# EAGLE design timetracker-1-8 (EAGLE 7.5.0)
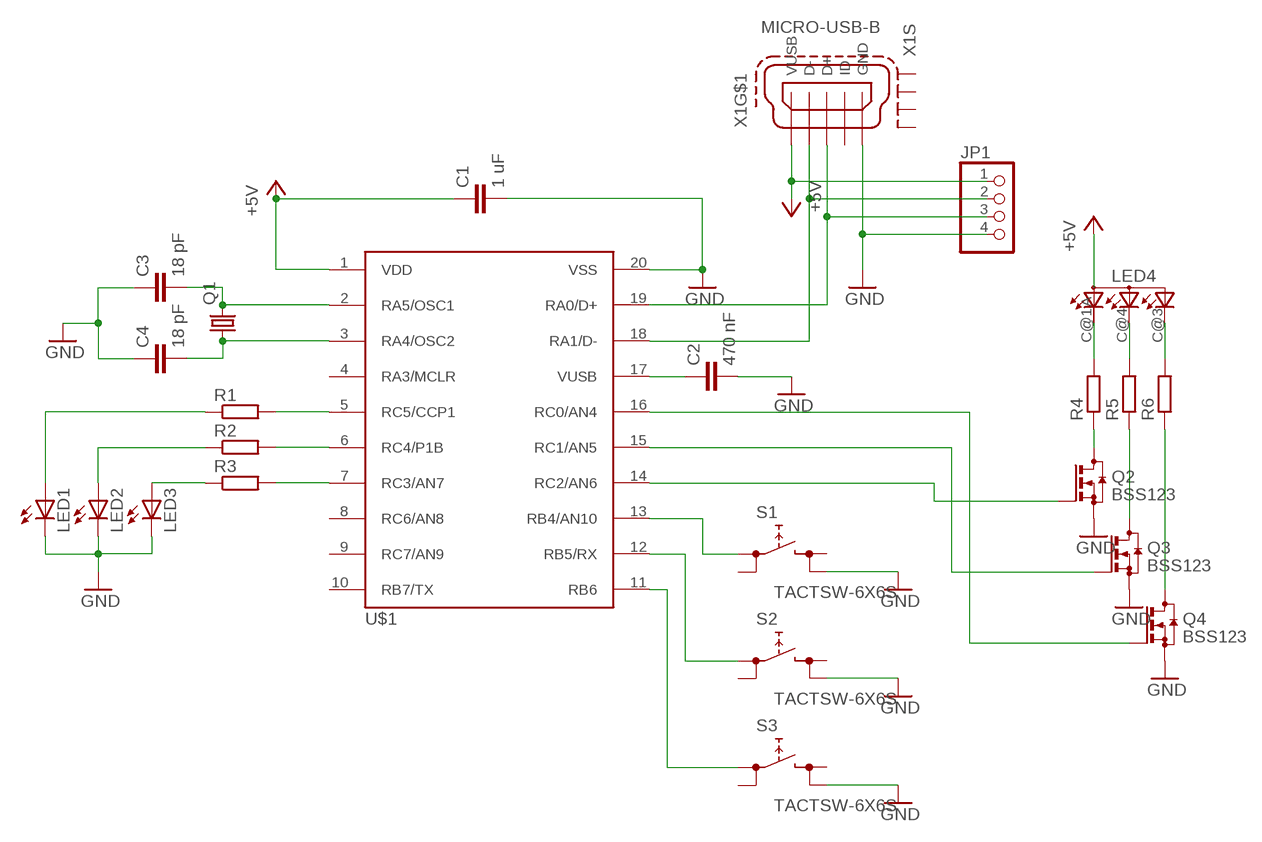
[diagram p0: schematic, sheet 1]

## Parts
C1  1 uF  C-EUC0805  [C0805]
C2  470 nF  C-EUC0805  [C0805]
C3  18 pF  C-EUC0805  [C0805]
C4  18 pF  C-EUC0805  [C0805]
JP1  PINHD-1X4  [1X04]
LED1  LEDSML0805  [SML0805]
LED2  LEDSML0805  [SML0805]
LED3  LEDSML0805  [SML0805]
LED4  RGBLED-3P-LCC-4  [P-LCC-4]
Q1  CRYSTALHC49UP  [HC49UP]
Q2  BSS123  [SOT23]
Q3  BSS123  [SOT23]
Q4  BSS123  [SOT23]
R1  R-EU_R0805  [R0805]
R2  R-EU_R0805  [R0805]
R3  R-EU_R0805  [R0805]
R4  R-EU_R0805  [R0805]
R5  R-EU_R0805  [R0805]
R6  R-EU_R0805  [R0805]
S1  TACTSW-6X6S  [TACTSW-6X6]
S2  TACTSW-6X6S  [TACTSW-6X6]
S3  TACTSW-6X6S  [TACTSW-6X6]
U$1  PIC18F14K50SMD  [DIL20-SMD]
X1  MICRO-USB-B  [MICRO-B-PAC]

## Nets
+5V: C1.1 JP1.1 LED4.A(A2) U$1.1(VDD) X1.1(VUSB)
GND: C1.2 C2.2 C3.1 C4.1 JP1.4 LED1.C LED2.C LED3.C Q2.2(S) Q3.2(S) Q4.2(S) S1.4(2.2) S2.4(2.2) S3.4(2.2) U$1.20(VSS) X1.5(GND)
N$1: JP1.3 U$1.19(RA0/D+) X1.3(D+)
N$2: C3.2 Q1.2 U$1.2(RA5/OSC1)
N$3: C2.1 U$1.17(VUSB)
N$4: C4.2 Q1.1 U$1.3(RA4/OSC2)
N$5: JP1.2 U$1.18(RA1/D-) X1.2(D-)
N$6: R3.2 U$1.7(RC3/AN7)
N$7: R2.2 U$1.6(RC4/P1B)
N$8: R1.2 U$1.5(RC5/CCP1)
N$9: LED1.A R1.1
N$10: LED2.A R2.1
N$11: LED3.A R3.1
N$12: LED4.C@1(CRED) R4.2
N$13: LED4.C@4(CGREEN) R5.2
N$14: S1.1(1.1) U$1.13(RB4/AN10)
N$15: S2.1(1.1) U$1.12(RB5/RX)
N$16: LED4.C@3(CBLUE) R6.2
N$17: Q2.3(D) R4.1
N$18: Q3.3(D) R5.1
N$19: Q4.3(D) R6.1
N$20: Q4.1(G) U$1.16(RC0/AN4)
N$21: Q3.1(G) U$1.15(RC1/AN5)
N$22: Q2.1(G) U$1.14(RC2/AN6)
N$23: S3.1(1.1) U$1.11(RB6)
Unconnected: S1.2(1.2) S1.3(2.1) S2.2(1.2) S2.3(2.1) S3.2(1.2) S3.3(2.1) U$1.4(RA3/MCLR) U$1.8(RC6/AN8) U$1.9(RC7/AN9) U$1.10(RB7/TX) X1.4(ID) X1.M1(S:S1) X1.M2(S:S2) X1.M3(S:S3) X1.M4(S:S4)

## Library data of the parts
C1-C4 = rcl:C-EU: CAPACITOR, European symbol
JP1 = pinhead:PINHD-1X4: PIN HEADER
LED1-LED3 = led:LED: LED
LED4 = g-e2e-training:RGBLED-3: OSRAM - Hyper Multi TOPLED® (RGB) LB E673, LV E673, LT E673 - Power TOPLED® Enhanced optical Power LED (HOP2000) LS E67B, LA E67B, LO E67B, LY E67B - Hyper Multi TOPLED® Enhanced optical Power LED (HOP2000 / ATON®) LATB T66B - Hyper Multi TOPLED® Hyper-Bright LED LATB T686 Source: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
Q1 = g-e2e-training:CRYSTAL: CRYSTAL; OC_FARNELL: unknown; OC_NEWARK: unknown
Q2-Q4 = transistor-small-signal:BSS123: N-CHANNEL MOS FET
R1-R6 = rcl:R-EU_: RESISTOR, European symbol
S1-S3 = g-e2e-training:TACTSW-6X6: 6.2 X 6.5mm TACT Switch (SMD) Source: http://www3.alps.co.jp/WebObjects/catalog.woa/PDF/E/Switch/Tact/SKHM/SKHM.PDF
U$1 = pic18f14k50:PIC18F14K50
X1 = g-e2e-training:MICRO-USB-B: MINI USB-B Conector Source: www.cypressindustries.com

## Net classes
0 default: width 0.305 mm

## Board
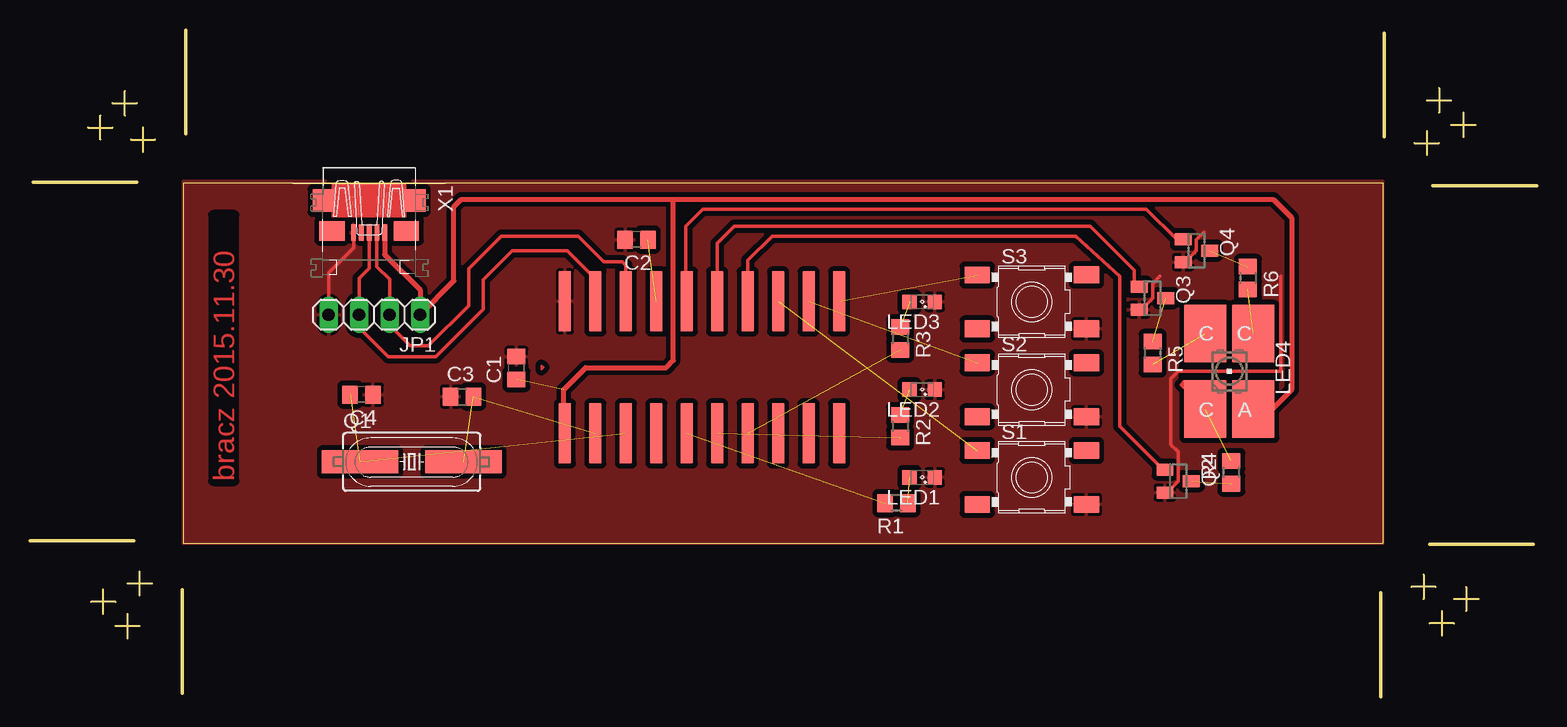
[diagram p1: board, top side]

Size 125.55 x 55.55 mm. Coordinates in mm from the lower left corner, seen from the top.
Outline: 36 segments
Copper layers (1*16): Top 0.035mm / dielectric 1.5mm / Bottom 0.035mm
Design rules "default *": minimum track width 10mil, minimum drill 24mil, track to track 12mil, track to pad 12mil, pad to pad 8mil, via to via 8mil, smd to smd 8mil, copper to edge 0mil, drill to drill 8mil, minimum pad ring 10mil, minimum via ring 8mil, stop-mask expansion 4mil, vias tented up to drill 0mil, thermal gap 10mil

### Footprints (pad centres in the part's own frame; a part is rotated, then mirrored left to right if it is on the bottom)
C0805 = smd 1.3 x 1.5: 1 -0.95,0; 2 0.95,0
1X04 = drill 1.016 long: 1 -3.81,0; 2 -1.27,0; 3 1.27,0; 4 3.81,0
SML0805 = smd 1.2 x 1.2: A 1.05,0; C -1.05,0
P-LCC-4 = smd 3.5 x 4.8: A -2,3.15; C@1 2,3.15; C@3 -2,-3.15; C@4 2,-3.15
HC49UP = smd 6.35 x 1.93: 1 -4.318,0; 2 4.318,0
SOT23 = smd 1 x 1.4: 1 -0.95,-1.1; 2 0.95,-1.1; 3 0,1.1
R0805 = smd 1.3 x 1.5: 1 -0.95,0; 2 0.95,0
TACTSW-6X6 = smd 2.1 x 1.4: 1 -4.55,2.24; 2 4.55,2.25; 3 -4.55,-2.25; 4 4.55,-2.25
DIL20-SMD = smd 1 x 5: 1 -11.43,-5.5; 2 -8.89,-5.5; 3 -6.35,-5.5; 4 -3.81,-5.5; 5 -1.27,-5.5; 6 1.27,-5.5; 7 3.81,-5.5; 8 6.35,-5.5; 9 8.89,-5.5; 10 11.43,-5.5; 11 11.43,5.5; 12 8.89,5.5; 13 6.35,5.5; 14 3.81,5.5; 15 1.27,5.5; 16 -1.27,5.5; 17 -3.81,5.5; 18 -6.35,5.5; 19 -8.89,5.5; 20 -11.43,5.5
MICRO-B-PAC = smd 1.35 x 0.4: 1 2.675,1.3; 2 2.675,0.65; 3 2.675,0; 4 2.675,-0.65; 5 2.675,-1.3 | smd 1.9 x 1.8: M1 0,-3.8; M2 0,3.8 | smd 1.6 x 2.1: M3 2.55,3.1; M4 2.55,-3.1

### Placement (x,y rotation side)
C1  40.54,27.38 90 top
C2  50.54,38.08 180 top
C3  36,24.99 0 top
C4  27.63,25.17 180 top
JP1  28.69,31.82 180 top
LED1  74.34,18.26 180 top
LED2  74.34,25.58 180 top
LED3  74.34,32.89 180 top
LED4  99.95,27.1 180 top
Q1  31.81,19.56 0 top
Q2  95.68,17.96 270 top
Q3  93.55,33.2 270 top
Q4  97.2,37.16 270 top
R1  72.21,16.13 180 top
R2  72.51,22.53 270 top
R3  72.51,29.84 270 top
R4  100.12,18.69 90 top
R5  93.55,28.62 270 top
R6  101.5,34.88 270 top
S1  83.49,18.26 0 top
S2  83.49,25.58 0 top
S3  83.49,32.89 0 top
U$1  56,27.43 0 top
X1  28.26,41.34 270 top

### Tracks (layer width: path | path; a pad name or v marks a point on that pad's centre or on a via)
+5V  (1 unrouted)
  Top 0.406: X1.1 29.56,36.83 32.5,33.89 JP1.1 35.33,34.65 35.33,40.82 35.94,41.42 53.62,41.42 | 53.62,41.42 103.6,41.42 105.13,39.9 105.13,25.58 103.54,23.99 LED4.A | U$1.1 44.47,22.03 44.47,25.58 46.3,27.4 53.01,27.4 53.62,28.01 53.62,41.42
GND
  Top 0.305: X1.5 26.96,37.4 24.88,35.32 JP1.4 | Q4.2 96.25,36.21 97.2,37.16 97.2,38.07 97.81,38.68 | Q3.2 92.6,32.25 93.55,33.2 93.55,34.41 94.16,35.02 | Q2.2 94.73,17.01 95.68,17.96 95.68,20.39 95.07,21 95.07,26.49 95.68,27.1 104.21,27.1 104.21,35.02
  pour Top (isolate 0.406): 12.77,42.64 12.77,12.77 112.75,12.77 112.75,42.95 12.77,42.95
N$1
  Top 0.305: X1.3 28.26,35.7 27.42,34.86 JP1.3 27.4,31.8 27.4,30.76 29.84,28.32 33.8,28.32 37.77,32.28 37.77,34.72 40.21,37.16 44.78,37.16 47.11,34.83 U$1.19
N$2  (2 unrouted)
N$3  (1 unrouted)
N$4  (2 unrouted)
N$5
  Top 0.305: X1.2 28.91,35.81 29.96,34.76 JP1.2 29.96,30.94 31.67,29.23 33.2,29.23 36.55,32.59 36.55,35.63 39.29,38.38 45.69,38.38 47.83,36.24 49.35,36.24 49.65,35.94 U$1.18
N$6  (1 unrouted)
N$7  (1 unrouted)
N$8  (1 unrouted)
N$9  (1 unrouted)
N$10  (1 unrouted)
N$11  (1 unrouted)
N$12  (1 unrouted)
N$13  (1 unrouted)
N$14  (1 unrouted)
N$15  (1 unrouted)
N$16  (1 unrouted)
N$17  (1 unrouted)
N$18  (1 unrouted)
N$19  (1 unrouted)
N$20
  Top 0.305: U$1.16 54.63,33.03 54.63,39.19 56.06,40.61 93.04,40.61 95.54,38.11 Q4.1
N$21
  Top 0.305: Q3.1 92.02,34.57 92.02,35.53 88.36,39.19 58.7,39.19 57.27,37.76 U$1.15
N$22
  Top 0.305: Q2.1 94.42,18.91 90.8,22.53 90.8,35.02 87.14,38.38 61.85,38.38 59.81,36.34 U$1.14
N$23  (1 unrouted)

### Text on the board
Top: bracz 2015.11.30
